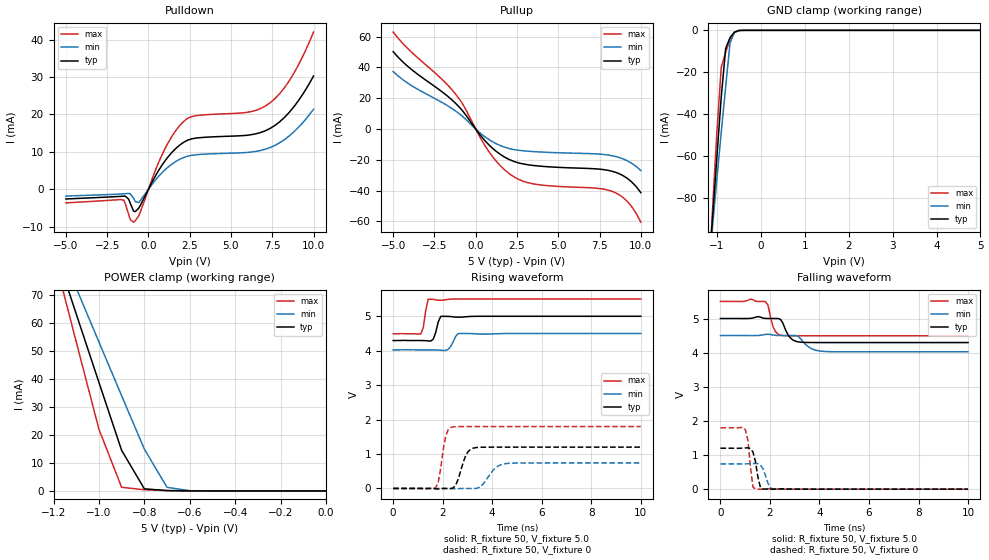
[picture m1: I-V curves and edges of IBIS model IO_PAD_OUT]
[IBIS Ver]   3.2
[Comment Char]   |_char
[File name]   sg-3031cma_5v_.ibs
[File Rev]   1.0
[Date]   2019/09/27 16:41:15
[Source]
[Notes]
[Disclaimer]
This information is for modeling purposes only, and is not guaranteed.
Property of SEIKO EPSON Corp.,
unauthorized reproduction and/or distribution is strictly prohibited.
[Copyright]
Copyright 2019, SEIKO EPSON Corp.
[Component]   G9T010W0A
Si_location Pin
Timing_location Pin
[Manufacturer]   SEIKO EPSON Corp.
| SG-3031CMA
[Package]
R_pkg   0.0m   0.0m   0.0m
L_pkg   0.0n   0.0n   0.0n
C_pkg   0.0p   0.0p   0.0p
[Pin] signal_name   model_name
1   VIO   POWER
2   GND   GND
3   OUT   IO_PAD_OUT
4   Vcc   POWER
| Models and submodels in the file (1): IO_PAD_OUT (3-state)
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[Model]   IO_PAD_OUT
Model_type 3-state
Enable Active-High
Polarity Non-Inverting
Vmeas=2.50
C_comp   2.5p   2.0p   3.0p
[Temperature Range] 25   105   -40
[Voltage Range]   5.0   4.5   5.5
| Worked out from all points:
|   slope of the pulldown table from 0 to 0.75 V, typ, clamps not added: 126 ohm
|   slope of the pullup table from 0 to 0.75 V, typ, clamps not added: 77.2 ohm
|   GND clamp passes 1 mA (typ) near -0.61 V on its own axis
|   POWER clamp passes 1 mA (typ) near -0.80 V on its own axis
|   falling waveform, R_fixture 50, V_fixture 5.0: 20-80 % time 297ps typ, 432ps min, 222ps max; typ from 5 V to 4.29 V
|   falling waveform, R_fixture 50, V_fixture 0: 20-80 % time 191ps typ, 218ps min, 155ps max; typ from 1.2 V to 0 V
|   rising waveform, R_fixture 50, V_fixture 5.0: 20-80 % time 165ps typ, 197ps min, 136ps max; typ from 4.29 V to 5 V
|   rising waveform, R_fixture 50, V_fixture 0: 20-80 % time 324ps typ, 469ps min, 237ps max; typ from 0 V to 1.2 V
[Pullup]
-5V       50.26mA    37.36mA    62.97mA
-3.9V     38.78mA    28.31mA    50.07mA
-2.1V     24.67mA    17.62mA    32.86mA
-1.2V     16.51mA    11.59mA    22.44mA
-800mV    11.88mA    8.23mA     16.39mA
800mV     -10.27mA   -6.822mA   -14.69mA
2V        -19.62mA   -12.59mA   -28.7mA
2.7V      -22.26mA   -13.92mA   -33.16mA
3.5V      -23.66mA   -14.65mA   -35.61mA
8.3V      -27.53mA   -17.42mA   -40.62mA
9.2V      -32.18mA   -20.74mA   -47.2mA
10V       -41.31mA   -26.95mA   -60.49mA
[Pulldown]
-5V       -2.593mA   -1.813mA   -3.63mA
-1.5V     -1.851mA   -1.212mA   -2.889mA
-1.1V     -3.744mA   -1.21mA    -8.132mA
-900mV    -5.848mA   -2.398mA   -8.803mA
-600mV    -5.116mA   -3.564mA   -7.202mA
900mV     6.952mA    4.772mA    9.936mA
2V        12.16mA    8.239mA    17.55mA
2.7V      13.56mA    9.131mA    19.52mA
6.1V      14.52mA    9.9mA      20.68mA
7.3V      16.11mA    11.05mA    22.9mA
8.6V      20.93mA    14.53mA    29.51mA
10V       30.28mA    21.4mA     42.04mA
[GND Clamp]
-5V       -1.289A    -1.043A    -1.612A
-1.2V     -119.6mA   -117.1mA   -123.7mA
-1.1V     -89.89mA   -93.84mA   -85.78mA
-1V       -60.43mA   -70.87mA   -48.68mA
-900mV    -31.78mA   -48.53mA   -17.64mA
-800mV    -8.711mA   -27.01mA   -10.46mA
-700mV    -3.454mA   -6.09mA    -4.512mA
-600mV    -868.8uA   -934.6uA   -956.3uA
-500mV    -86.23uA   -135.8uA   -52.66uA
-400mV    -4.725uA   -14.7uA    -1.074uA
5V        58.37pA    6.372uA    34.13pA
[POWER Clamp]
-5V       1.033A     837.7mA    1.291A
-1.2V     87.99mA    92.06mA    84.88mA
-1.1V     63.39mA    72.67mA    53.41mA
-1V       38.88mA    53.35mA    22.1mA
-900mV    14.55mA    34.1mA     1.304mA
-800mV    762.8uA    15mA       407.8uA
-700mV    113uA      1.289mA    132.2uA
-600mV    21.58uA    79.3uA     21.07uA
0V        58.37pA    1.101nA    44.71pA
[Falling Waveform]
R_fixture=50
V_fixture=5.0
V_fixture_min=4.5
V_fixture_max=5.5
0s        5V         4.5V       5.5V
1.818ns   5.002V     4.534V     5.494V
1.919ns   5V         4.539V     5.396V
2.222ns   5V         4.506V     4.616V
2.525ns   4.858V     4.5V       4.501V
2.828ns   4.429V     4.5V       4.492V
3.232ns   4.307V     4.412V     4.492V
3.636ns   4.296V     4.132V     4.492V
4.141ns   4.295V     4.038V     4.492V
10ns      4.295V     4.024V     4.492V
[Falling Waveform]
R_fixture=50
V_fixture=0
V_fixture_min=0
V_fixture_max=0
0s        1.2V       740.9mV    1.798V
1.01ns    1.208V     740.8mV    1.74V
1.111ns   1.212V     743.2mV    1.424V
1.313ns   1.089V     750mV      60.52mV
1.414ns   811.2mV    751.7mV    4.361mV
1.616ns   48.5mV     705.3mV    170.3uV
1.717ns   6.473mV    598.7mV    382.1uV
1.919ns   268.7uV    173.3mV    12.74mV
2.121ns   131.9uV    8.321mV    5.314mV
10ns      0V         0V         -1.511uV
[Rising Waveform]
R_fixture=50
V_fixture=5.0
V_fixture_min=4.5
V_fixture_max=5.5
0s        4.295V     4.024V     4.492V
1.111ns   4.295V     4.024V     4.483V
1.212ns   4.295V     4.024V     4.661V
1.313ns   4.291V     4.024V     5.16V
1.414ns   4.283V     4.024V     5.495V
1.616ns   4.335V     4.024V     5.493V
1.919ns   4.996V     4.013V     5.463V
2.222ns   4.996V     4.043V     5.493V
2.626ns   4.973V     4.495V     5.5V
10ns      5V         4.5V       5.5V
[Rising Waveform]
R_fixture=50
V_fixture=0
V_fixture_min=0
V_fixture_max=0
0s        0V         0V         0V
1.717ns   -10.68mV   102.2uV    24.09mV
1.818ns   -17.97mV   220.4uV    178.4mV
2.121ns   -1.922mV   -573.8uV   1.521V
2.424ns   14.99mV    -9.726mV   1.787V
2.626ns   270.5mV    -7.876mV   1.796V
2.929ns   955.5mV    -1.205mV   1.797V
3.232ns   1.17V      -3.48mV    1.798V
4.545ns   1.2V       720mV      1.798V
10ns      1.2V       740.9mV    1.798V
[Ramp]
R_load=50
dV/dt_r   7.199E-1/3.192E-10   4.445E-1/4.640E-10   1.079E+0/2.235E-10
dV/dt_f   4.228E-1/2.934E-10   2.856E-1/4.280E-10   6.049E-1/2.176E-10
|[End   IO_PAD_OUT
